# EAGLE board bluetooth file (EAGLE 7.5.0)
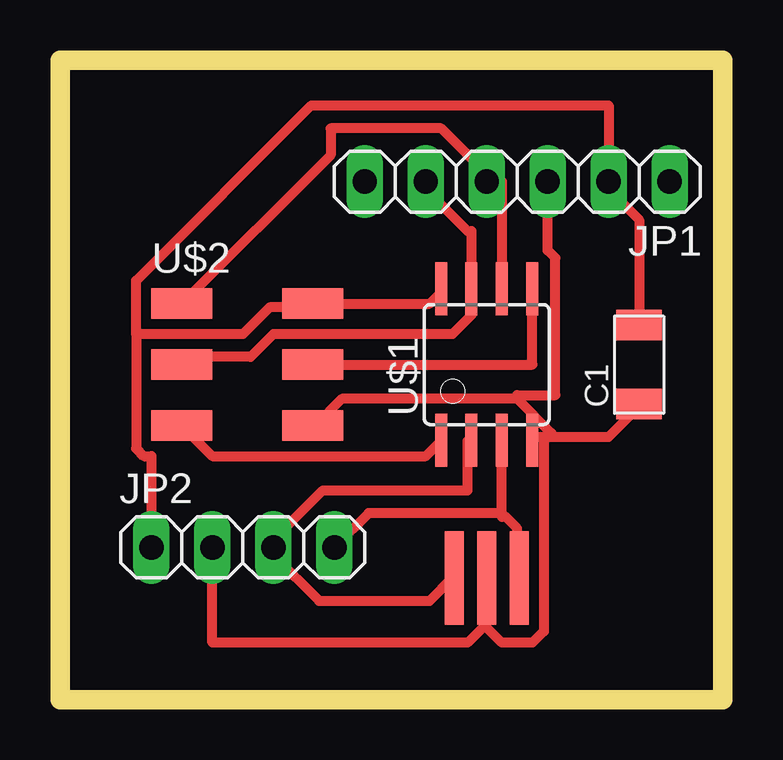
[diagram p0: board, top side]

Size 27.61 x 26.66 mm. Coordinates in mm from the lower left corner, seen from the top.
Outline: 0,0 27.61,0 27.61,26.66 0,26.66 0,0
Copper layers (1*16): Top 0.035mm / dielectric 1.5mm / Bottom 0.035mm
Design rules "default *": minimum track width 16mil, minimum drill 24mil, track to track 16mil, track to pad 16mil, pad to pad 16mil, via to via 8mil, smd to smd 16mil, copper to edge 40mil, drill to drill 8mil, minimum pad ring 10mil, minimum via ring 8mil, stop-mask expansion 4mil, vias tented up to drill 0mil, thermal gap 10mil

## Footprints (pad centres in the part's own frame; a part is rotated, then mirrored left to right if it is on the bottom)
C1206FAB = smd 1.27 x 1.905: 1 -1.651,0; 2 1.651,0
1X06 = drill 1.016 long: 1 -6.35,0; 2 -3.81,0; 3 -1.27,0; 4 1.27,0; 5 3.81,0; 6 6.35,0
1X04 = drill 1.016 long: 1 -3.81,0; 2 -1.27,0; 3 1.27,0; 4 3.81,0
SOIC8 = smd 0.5 x 2.2: 1 -1.905,-3.154; 2 -0.645,-3.154; 3 0.625,-3.154; 4 1.895,-3.154; 5 1.905,3.154; 6 0.635,3.154; 7 -0.635,3.154; 8 -1.905,3.154
2X03SMD = smd 2.54 x 1.27: 1 -2.54,2.54; 2 2.92,2.54; 3 -2.54,0; 4 2.92,0; 5 -2.54,-2.54; 6 2.92,-2.54
EFOBM = smd 0.8 x 3.9: 1 -1.35,0; 2 0,0; 3 1.35,0

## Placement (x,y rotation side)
C1  [C1206FAB]  24.13,13.97 90 top
JP1  [1X06]  19.05,21.59 180 top
JP2  [1X04]  7.62,6.35 0 top
U$1  ATTINY45SI  [SOIC8]  17.78,13.97 0 top
U$2  AVRISPSMD  [2X03SMD]  7.62,13.97 0 top
U$3  RESONATOR  [EFOBM]  17.78,5.08 180 top

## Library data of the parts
C1 U$1-U$3 = fab
JP1 JP2 = pinhead

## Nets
GND: C1.1 JP1.3 JP2.2 U$1.4 U$2.6 U$3.2
MOSI: U$1.5 U$2.4
N$1: JP1.1
N$5: JP2.3 U$1.2 U$3.3
N$6: JP1.6
N$7: JP2.4 U$1.3 U$3.1
RST: U$1.1 U$2.5
RX: JP1.5 U$1.7 U$2.3
TX: JP1.4 U$1.6 U$2.1
VCC: C1.2 JP1.2 JP2.1 U$1.8 U$2.2

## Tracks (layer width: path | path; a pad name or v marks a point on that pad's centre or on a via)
GND
  Top 0.406: JP2.2 6.35,2.38 16.99,2.38 17.7,3.1 | 17.7,3.1 17.78,3.17 U$3.2 | 20.16,10.95 19.69,10.95 U$1.4 | 20.16,10.95 20.48,10.95 | 20.48,10.95 22.86,10.95 24.13,12.22 C1.1 | 19.05,12.54 11.75,12.54 10.64,11.43 U$2.6 | 19.05,12.54 20.48,11.11 20.48,10.95 | JP1.3 20.32,18.73 20.64,18.41 20.64,12.7 19.05,12.7 19.05,12.54 | 17.7,3.1 18.41,2.38 19.69,2.38 20.16,2.86 20.16,10.95
MOSI
  Top 0.406: U$1.5 19.69,13.97 U$2.4
N$5
  Top 0.406: U$1.2 16.99,10.8 16.99,8.73 10.95,8.73 8.89,6.67 JP2.3 8.89,6.03 10.8,4.13 15.4,4.13 16.35,5.08 U$3.3
N$7
  Top 0.406: 18.41,7.78 18.41,7.62 18.57,7.62 19.05,7.14 19.05,5.08 U$3.1 | 18.41,7.78 18.41,10.8 U$1.3 | JP2.4 12.86,7.78 18.41,7.78
RST
  Top 0.406: U$2.5 6.35,10.16 15.24,10.16 15.88,10.8 U$1.1
RX
  Top 0.406: JP1.5 15.24,21.27 16.99,19.53 17.15,19.53 U$1.7 17.15,16.03 16.35,15.24 8.89,15.24 7.94,14.29 5.4,14.29 U$2.3
TX
  Top 0.406: U$1.6 18.41,21.59 JP1.4 17.94,21.75 15.88,23.81 11.27,23.81 11.27,22.7 U$2.1
VCC
  Top 0.406: C1.2 24.13,20 22.86,21.27 JP1.2 22.86,24.77 10.48,24.77 3.18,17.46 3.18,15.24 | U$1.8 15.88,16.99 15.4,16.51 U$2.2 10.48,16.35 8.73,16.35 7.62,15.24 3.18,15.24 | JP2.1 3.81,10.16 3.49,10.16 3.18,10.48 3.18,15.24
